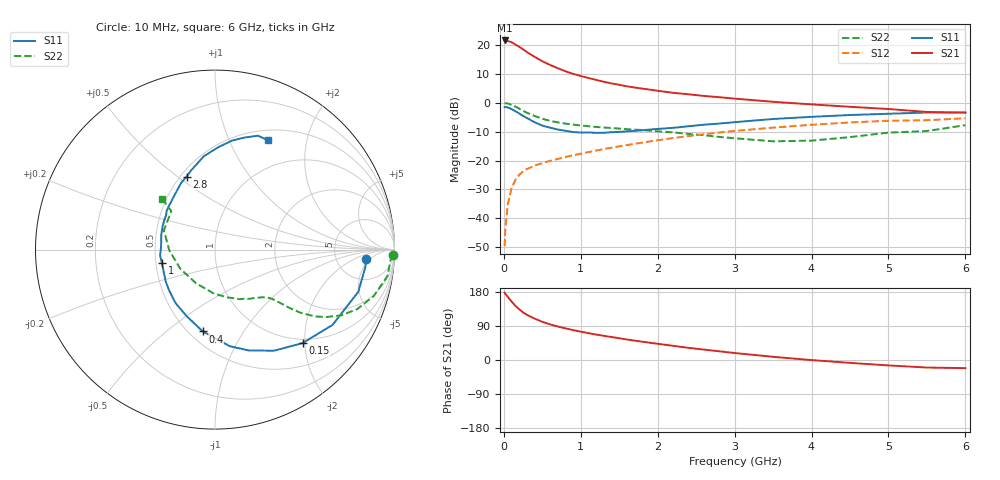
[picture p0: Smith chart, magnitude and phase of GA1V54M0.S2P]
! Infineon Technologies  Discrete & RF Semiconductors
! BF775
! Si NPN RF Bipolar Junction Transistor in SOT23
! VCE = 1.5 V  IC = 4 mA
! Common Emitter S-Parameters:  May  1996
# GHz  S  MA  R  50
!  f  S11  S21  S12  S22
! GHz  MAG  ANG  MAG  ANG  MAG  ANG  MAG  ANG
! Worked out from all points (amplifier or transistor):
!   36 points, 10 MHz to 6 GHz, reference 50 ohm
!   highest |S21| = 21.6 dB at 10 MHz (marker M1)
!   |S21| within 3 dB of that: start of sweep to 245.7 MHz
!   unconditionally stable (mu >= 1): 829.1 MHz to 4.457 GHz; 5.046 GHz to end of sweep
!   at 250 MHz: K = 0.44, MSG = 21.1 dB, |S12| = -23.8 dB
!   at 1.4 GHz: K = 1.15, MAG = 8.7 dB, |S12| = -15.5 dB
!   at 6 GHz: K = 1.01, MAG = 0.3 dB, |S12| = -5.4 dB
!   S11 on the Smith chart (normalised r, x): 10 MHz: 10, -4; 150 MHz: 0.92, -1.95; 400 MHz: 0.58, -0.68; 1 GHz: 0.54, -0.09; 2.8 GHz: 0.54, +0.54; 6 GHz: 0.62, +1.40
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0.01  0.8422 -3.7  11.97 177.5  0.0033 88.2  0.9917 -1.7
0.02  0.8437 -6.5  11.8 174.5  0.0068 87.2  0.9794 -3.5
0.05  0.8324 -16.4  11.71 166.8  0.0173 82.3  0.9725 -8.7
0.1  0.7775 -32.7  11.18 154.5  0.0334 72.8  0.9211 -16.4
0.15  0.7135 -46.9  10.17 143.0  0.0464 65.7  0.8578 -22.8
0.2  0.6525 -59.7  9.317 133.7  0.0566 61.1  0.7918 -27.6
0.25  0.593 -71.4  8.402 125.6  0.0647 57.2  0.725 -31.2
0.3  0.5445 -81.3  7.529 119.3  0.0712 54.9  0.6716 -33.7
0.4  0.4609 -98.5  6.231 109.3  0.0817 51.6  0.5911 -36.5
0.5  0.4031 -113.1  5.226 100.7  0.0904 50.7  0.5286 -38.0
0.6  0.371 -126.1  4.519 94.1  0.0985 50.5  0.4865 -38.9
0.8  0.3276 -146.8  3.516 83.5  0.1151 50.6  0.436 -40.2
1  0.305 -165.7  2.901 74.8  0.1313 51.1  0.4048 -41.8
1.1  0.3075 -173.7  2.681 70.9  0.14 51.4  0.3925 -43.1
1.3  0.3022 172.6  2.31 63.8  0.1584 51.6  0.3727 -45.5
1.6  0.3205 155.3  1.925 54.0  0.1854 50.9  0.3493 -50.4
2.2  0.3682 130.0  1.487 37.4  0.2446 47.3  0.3079 -63.8
2.8  0.4366 111.3  1.248 23.0  0.3056 41.8  0.2564 -83.5
3.5  0.5239 96.8  1.04 8.4  0.3716 33.4  0.2154 -119.2
4.5  0.6139 81.2  0.852 -7.6  0.4561 20.2  0.2547 -179.0
5.5  0.6782 69.3  0.693 -19.9  0.4984 5.8  0.3242 138.7
6  0.6766 64.2  0.675 -21.5  0.5397 1.8  0.4096 136.1
